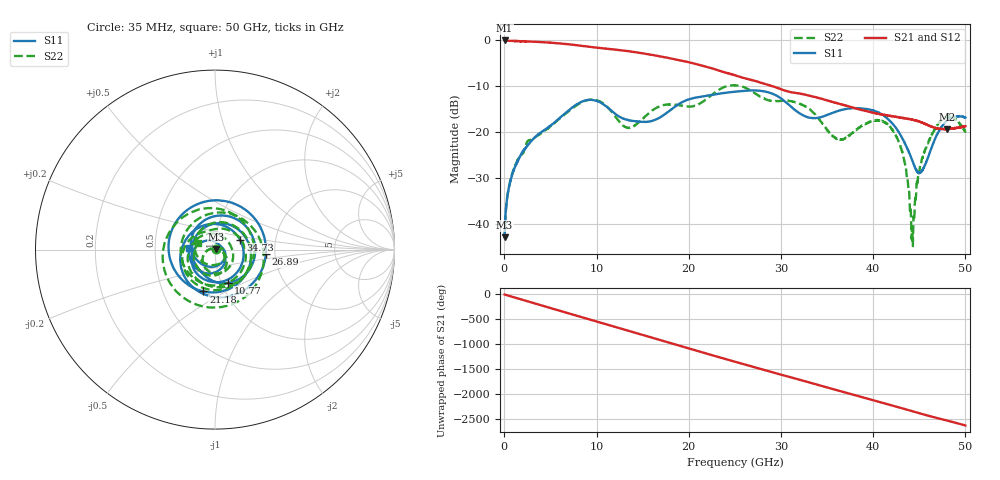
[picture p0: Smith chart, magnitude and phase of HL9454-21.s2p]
! 3/7/2022 11:46:20 AM
! H:\PRODUCTION_DATA\TEMP_S2P.S2P
! CHANNEL.1
! TR.MEASUREMENT
! CORRECTED.DATA
# GHZ S RI R 50.0
! FREQ.GHZ  S11RE  S11IM  S21RE  S21IM  S12RE  S12IM  S22RE  S22IM
!; PortSelection: Port_12
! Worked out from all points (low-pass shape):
!   3571 points, 35 MHz to 50 GHz, reference 50 ohm
!   highest |S21| = -0.05 dB at 35 MHz (marker M1); lowest = -19.4 dB at 47.97 GHz (marker M2)
!   |S21| within 3 dB of the highest: start of sweep to 15.62 GHz
!   lowest |S11| = -42.9 dB at 35 MHz (marker M3), VSWR 1.01, Z = 50.6 + j0.338 ohm
!   |S11| at or under -10 dB: start of sweep to end of sweep
!   |S22| runs from -44.8 to -9.8 dB; largest |S21 - S12| = 0.0079
!   S11 on the Smith chart (normalised r, x): 35 MHz: 1.01, +0.01; 10.77 GHz: 1.08, -0.42; 21.18 GHz: 0.79, -0.39; 26.89 GHz: 1.79, -0.10; 34.73 GHz: 1.32, +0.14; 50 GHz: 0.75, +0.01
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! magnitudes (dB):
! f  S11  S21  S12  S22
! 35 MHz  -42.9  -0.1  -0.1  -42.7
! 398.9 MHz  -33.1  -0.1  -0.1  -33.1
! 832.8 MHz  -29.4  -0.1  -0.2  -29.3
! 2.512 GHz  -22.9  -0.3  -0.3  -22.0
! 8.376 GHz  -13.4  -1.2  -1.2  -13.5
! 10.77 GHz  -14.0  -1.8  -1.8  -13.8
! 13.48 GHz  -17.4  -2.4  -2.4  -19.1
! 16.7 GHz  -17.0  -3.4  -3.4  -14.5
! 21.18 GHz  -12.3  -5.4  -5.4  -13.8
! 25.03 GHz  -11.2  -7.7  -7.8  -9.8
! 26.89 GHz  -10.9  -8.7  -8.7  -11.2
! 33.36 GHz  -16.9  -12.2  -12.2  -15.5
! 34.73 GHz  -16.5  -12.9  -12.9  -18.7
! 36.49 GHz  -15.2  -13.9  -14.0  -21.6
! 39.7 GHz  -15.1  -15.6  -15.6  -17.8
! 41.69 GHz  -17.3  -16.4  -16.4  -18.5
! 43.31 GHz  -21.9  -17.0  -17.0  -25.6
! 44.25 GHz  -26.2  -17.3  -17.3  -41.7
! 44.91 GHz  -28.8  -17.6  -17.7  -28.9
! 45.47 GHz  -27.9  -18.1  -18.1  -24.6
! 47.97 GHz  -17.5  -19.4  -19.3  -16.7
! 50 GHz  -16.8  -18.7  -18.8  -19.9
